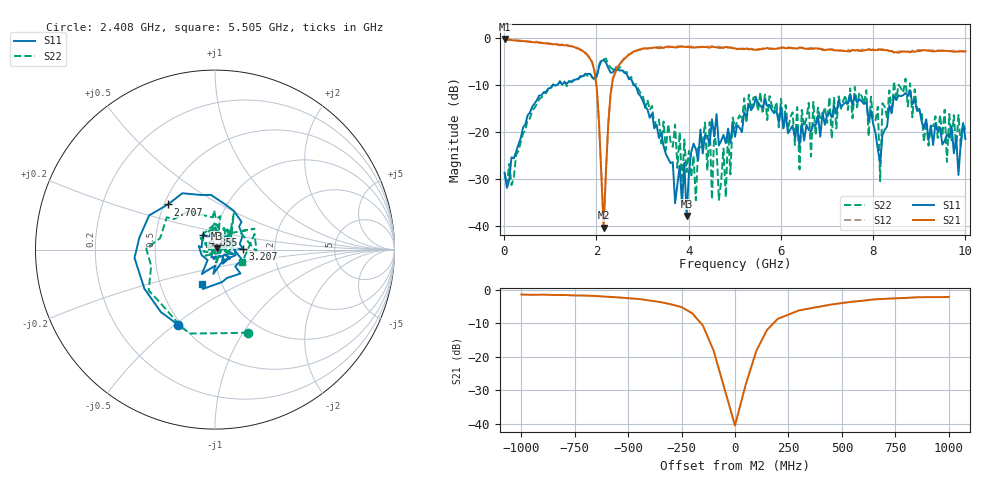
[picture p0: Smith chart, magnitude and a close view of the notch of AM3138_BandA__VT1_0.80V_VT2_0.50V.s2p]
! Date/Time: Tue, Nov 13, 2018 4:42 PM
! Network Analyzer: Agilent Technologies E8364B Rev: A.07.50.67
! Sweep from 0.010 to 10.000 GHz, 201 Points, Sweep Type: LIN
! Power Supply: 0.800 V, 0.000 A
# Hz S DB R 50
!freq MagS11 AngS11 MagS21 AngS21 MagS12 AngS12 MagS22 AngS22
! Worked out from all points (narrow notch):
!   201 points, 10 MHz to 10 GHz, reference 50 ohm
!   highest |S21| = -0.25 dB at 10 MHz (marker M1); lowest = -40.4 dB at 2.158 GHz (marker M2)
!   notch at M2: 38.1 dB deep, 170 MHz wide at half that depth
!   lowest |S11| = -38.0 dB at 3.956 GHz (marker M3), VSWR 1.03, Z = 51 + j0.73 ohm
!   |S11| at or under -10 dB: start of sweep to 1.055 GHz; 1.073 GHz to 1.159 GHz (86.01 MHz wide, 7.71 % of centre); 2.806 GHz to end of sweep
!   |S22| runs from -34.6 to -4.4 dB; largest |S21 - S12| = 0.027
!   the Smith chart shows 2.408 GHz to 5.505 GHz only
!   S11 on the Smith chart (normalised r, x): 2.408 GHz: 0.48, -0.52; 2.707 GHz: 0.52, +0.30; 3.207 GHz: 1.37, +0.01; 4.855 GHz: 0.86, +0.14; 5.505 GHz: 0.81, -0.33
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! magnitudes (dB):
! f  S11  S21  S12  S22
! 10 MHz  -28.7  -0.2  -0.3  -28.9
! 1.708 GHz  -8.1  -2.8  -2.7  -8.6
! 2.008 GHz  -8.2  -10.7  -10.7  -8.1
! 2.158 GHz  -4.7  -40.4  -39.9  -4.6
! 2.408 GHz  -6.6  -7.4  -7.4  -6.1
! 2.707 GHz  -8.8  -3.6  -3.4  -8.7
! 3.207 GHz  -16.1  -2.2  -2.1  -14.5
! 3.357 GHz  -21.3  -2.2  -1.9  -17.4
! 3.956 GHz  -38.0  -1.9  -1.8  -28.6
! 4.456 GHz  -22.6  -2.1  -1.9  -17.9
! 4.506 GHz  -17.3  -1.8  -1.8  -34.4
! 4.555 GHz  -21.0  -2.0  -1.9  -20.1
! 4.805 GHz  -22.4  -1.9  -1.8  -33.9
! 4.855 GHz  -19.3  -2.1  -2.0  -19.7
! 5.005 GHz  -21.1  -2.2  -2.1  -19.2
! 5.505 GHz  -13.7  -2.5  -2.4  -15.6
! 6.404 GHz  -22.8  -2.1  -2.0  -28.0
! 6.703 GHz  -18.4  -2.4  -2.2  -13.6
! 7.852 GHz  -13.6  -2.6  -2.6  -11.1
! 8.152 GHz  -26.7  -2.5  -2.3  -30.5
! 8.352 GHz  -14.3  -2.8  -2.8  -11.2
! 10 GHz  -21.5  -2.9  -2.7  -19.6
